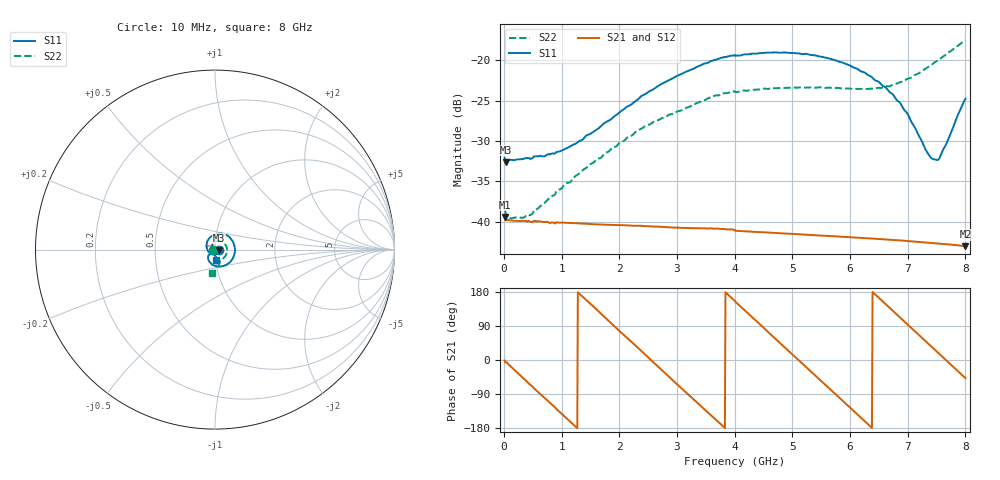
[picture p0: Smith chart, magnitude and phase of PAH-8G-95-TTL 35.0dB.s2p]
! MTS Systemtechnik GmbH
! S-Parameters
! Model: PAH-8G/95-TTL
! Attenuation Step: 35.0dB
! Rohde & Schwarz ZVB8 2Ports - Version 4.11 - 1145.1010k08 SN: 100119
! S2P File Measurements:
! S11 S21 S12 S22
# HZ  S  DB  R  50.00
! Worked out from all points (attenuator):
!   800 points, 10 MHz to 8 GHz, reference 50 ohm
!   highest |S21| = -39.39 dB at 10 MHz (marker M1); lowest = -43.0 dB at 8 GHz (marker M2)
!   lowest |S11| = -32.6 dB at 30 MHz (marker M3), VSWR 1.05, Z = 52.4 - j0.253 ohm
!   |S11| at or under -10 dB: start of sweep to end of sweep
!   |S22| runs from -39.5 to -17.6 dB; largest |S21 - S12| = 0.00016
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1e7  -32.10 -5.1  -39.39 -1.2  -39.30 -1.1  -38.58 -169.1
3e7  -32.60 -5.9  -39.80 -6.4  -39.81 -6.4  -39.07 -179.6
1.3e8  -32.31 -12.7  -39.82 -19.1  -39.82 -19.1  -39.55 177.2
4.6e8  -32.20 -44.8  -39.97 -65.7  -39.99 -65.4  -39.14 172.3
9e8  -31.39 -90.3  -40.06 -128.1  -40.06 -128.1  -36.30 162.9
1.35e9  -29.89 -136.7  -40.21 168.8  -40.21 168.8  -33.70 148.3
2.31e9  -24.90 144.5  -40.49 33.9  -40.47 33.9  -28.73 108.1
2.68e9  -23.16 119.5  -40.60 -18.8  -40.59 -18.5  -27.40 92.6
3.44e9  -20.54 72.3  -40.79 -124.7  -40.80 -125.1  -25.03 58.5
4.01e9  -19.47 36.4  -41.09 153.9  -41.09 153.8  -23.95 32.0
4.68e9  -19.04 -4.4  -41.36 59.6  -41.37 59.6  -23.48 2.4
5.34e9  -19.38 -45.0  -41.62 -32.8  -41.62 -32.8  -23.37 -25.4
5.73e9  -19.98 -69.2  -41.78 -87.5  -41.79 -87.6  -23.45 -39.8
6.11e9  -21.01 -93.3  -41.94 -141.2  -41.95 -141.2  -23.55 -51.6
6.36e9  -22.01 -108.6  -42.05 -176.3  -42.05 -176.4  -23.53 -57.7
6.67e9  -23.84 -126.0  -42.18 140.0  -42.19 140.0  -23.25 -63.8
6.86e9  -25.22 -135.0  -42.28 113.1  -42.29 113.1  -22.75 -67.5
6.99e9  -26.56 -138.6  -42.36 94.8  -42.36 94.7  -22.32 -69.8
7.37e9  -31.76 -127.5  -42.57 41.1  -42.57 41.1  -20.78 -77.6
7.49e9  -32.32 -110.9  -42.63 24.2  -42.64 24.2  -20.16 -80.7
7.57e9  -31.80 -101.5  -42.69 13.0  -42.69 12.9  -19.78 -83.1
8e9  -24.77 -84.4  -43.00 -47.7  -43.02 -47.6  -17.57 -98.1
